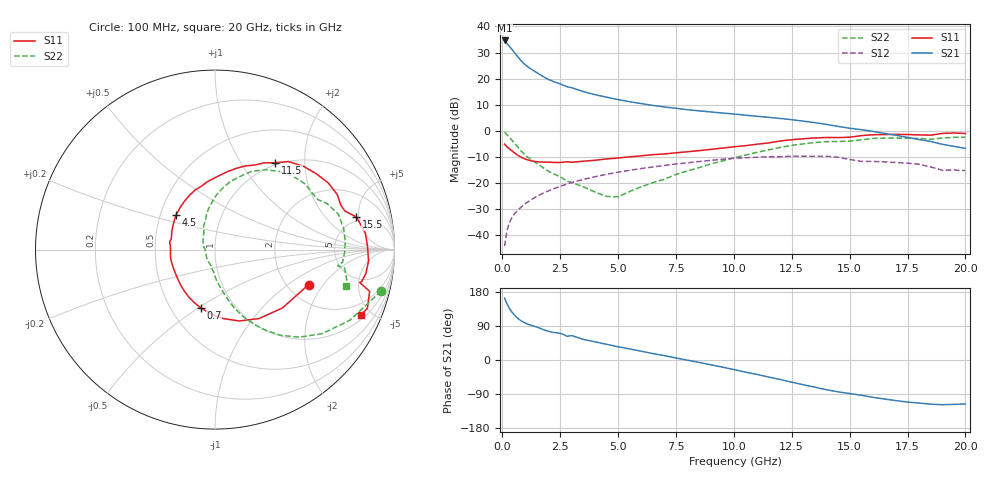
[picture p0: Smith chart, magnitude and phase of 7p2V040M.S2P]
! Infineon Technologies  Discrete & RF Semiconductors
! bfp620
! VCE =  2.0 V,  IC =  40 mA
! Common Emitter S-Parameters:  Sep 2002
# GHz  S  MA  R  50
!  f  S11  S21  S12  S22
! GHz  MAG  ANG  MAG  ANG  MAG  ANG  MAG  ANG
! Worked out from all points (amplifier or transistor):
!   59 points, 100 MHz to 20 GHz, reference 50 ohm
!   highest |S21| = 34.6 dB at 100 MHz (marker M1)
!   |S21| within 3 dB of that: start of sweep to 376.5 MHz
!   unconditionally stable (mu >= 1): 2.739 GHz to 9.841 GHz; 17.18 GHz to end of sweep
!   at 1 GHz: K = 0.82, MSG = 26.6 dB, |S12| = -27.9 dB
!   at 5.5 GHz: K = 1.04, MAG = 11.9 dB, |S12| = -15.1 dB
!   at 20 GHz: K = 1.27, MAG = 1.2 dB, |S12| = -15.2 dB
!   S11 on the Smith chart (normalised r, x): 100 MHz: 2.58, -1.46; 700 MHz: 0.70, -0.51; 4.5 GHz: 0.60, +0.25; 11.5 GHz: 0.97, +1.43; 15.5 GHz: 4.43, +4.66; 20 GHz: 1.23, -4.33
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0.1  0.5566 -20.6  53.82 163.3  0.0062 71.9  0.9543 -14.0
0.2  0.4966 -41.0  47.16 148.6  0.0122 71.3  0.8485 -27.6
0.3  0.4559 -57.4  41.84 137.0  0.0171 69.1  0.76 -38.0
0.4  0.42 -71.2  37.02 127.8  0.0212 67.1  0.6772 -46.1
0.5  0.3869 -83.2  32.59 120.3  0.0248 65.4  0.5997 -52.7
0.6  0.358 -94.1  28.63 113.9  0.0281 64.2  0.5295 -58.0
0.7  0.334 -103.8  25.23 108.5  0.0313 63.3  0.4686 -62.5
0.9  0.2998 -119.9  20.14 100.2  0.0374 62.4  0.3758 -69.2
1.1  0.2782 -131.9  16.88 94.7  0.0435 61.8  0.3145 -73.5
1.4  0.2597 -145.9  13.77 88.7  0.0527 60.8  0.2537 -78.0
1.8  0.2523 -162.2  10.75 79.6  0.0651 58.5  0.1919 -84.4
2.2  0.2494 -174.8  8.807 72.9  0.0774 55.9  0.1513 -89.5
2.8  0.2565 170.3  6.974 62.7  0.0961 51.3  0.1084 -99.0
3.5  0.2622 156.2  5.651 54.3  0.1177 45.2  0.0847 -110.5
4.5  0.2897 138.8  4.418 41.5  0.1473 36.1  0.0555 -155.7
7  0.3617 102.0  2.868 11.5  0.2178 12.2  0.1184 121.2
10.5  0.5201 64.9  1.999 -32.0  0.3067 -27.1  0.3438 83.0
11.5  0.588 55.4  1.816 -44.9  0.3199 -39.4  0.4322 70.9
13.5  0.732 30.6  1.436 -71.7  0.3268 -63.5  0.5969 43.4
15.5  0.8087 13.0  1.056 -93.0  0.2601 -85.6  0.6734 22.5
17  0.8577 -4.3  0.824 -107.2  0.2478 -95.4  0.7272 3.6
20  0.8902 -24.2  0.463 -116.1  0.1736 -105.1  0.7556 -15.7
